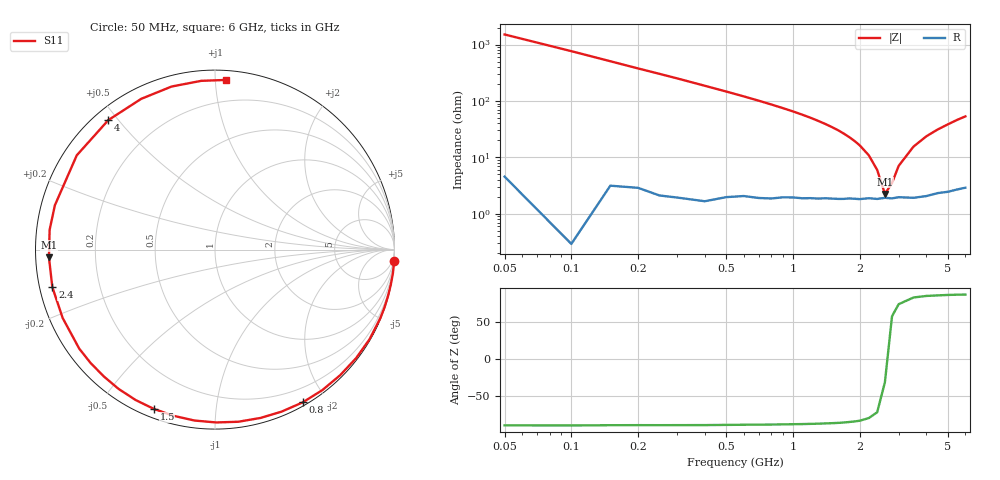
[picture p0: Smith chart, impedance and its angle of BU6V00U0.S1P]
! Infineon Technologies  Discrete & RF Semiconductors
! BB 833
! Si Tuning Diode in SOD323
! VR = 6 V
! S-Parameters:  June  1999
# GHz  S  MA  R  50
!  f  S11
! GHz  MAG  ANG
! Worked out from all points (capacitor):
!   34 points, 50 MHz to 6 GHz, reference 50 ohm
!   read as one part to ground: C = 2.09 pF near 50 MHz
!   lowest |Z| = 2.25 ohm at 2.6 GHz (marker M1)
!   series resonance near 2.657 GHz, so ESL is about 1.7 nH
!   S11 on the Smith chart (normalised r, x): 50 MHz: 0, -30; 800 MHz: 0.04, -1.73; 1.5 GHz: 0.04, -0.69; 2.4 GHz: 0.04, -0.11; 4 GHz: 0.04, +0.47; 6 GHz: 0.06, +1.06
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0.05  0.9998 -3.8
0.15  0.9988 -11.3
0.25  0.9978 -18.8
0.4  0.9955 -30.1
0.5  0.9918 -37.6
0.6  0.9879 -45.1
0.7  0.9851 -52.6
0.8  0.9814 -60.1
0.9  0.976 -67.6
1  0.9716 -74.9
1.1  0.9679 -82.3
1.2  0.9631 -89.6
1.3  0.9592 -96.9
1.5  0.9507 -111.0
1.6  0.9476 -117.8
1.8  0.9397 -131.3
2  0.9363 -143.9
2.2  0.9303 -155.8
2.4  0.9302 -167.0
2.6  0.9262 -177.3
2.8  0.928 173.2
3  0.9256 164.5
3.5  0.9323 145.7
4  0.9347 129.5
4.5  0.9352 116.1
5  0.9402 104.9
5.5  0.9433 94.7
6  0.9471 86.4
